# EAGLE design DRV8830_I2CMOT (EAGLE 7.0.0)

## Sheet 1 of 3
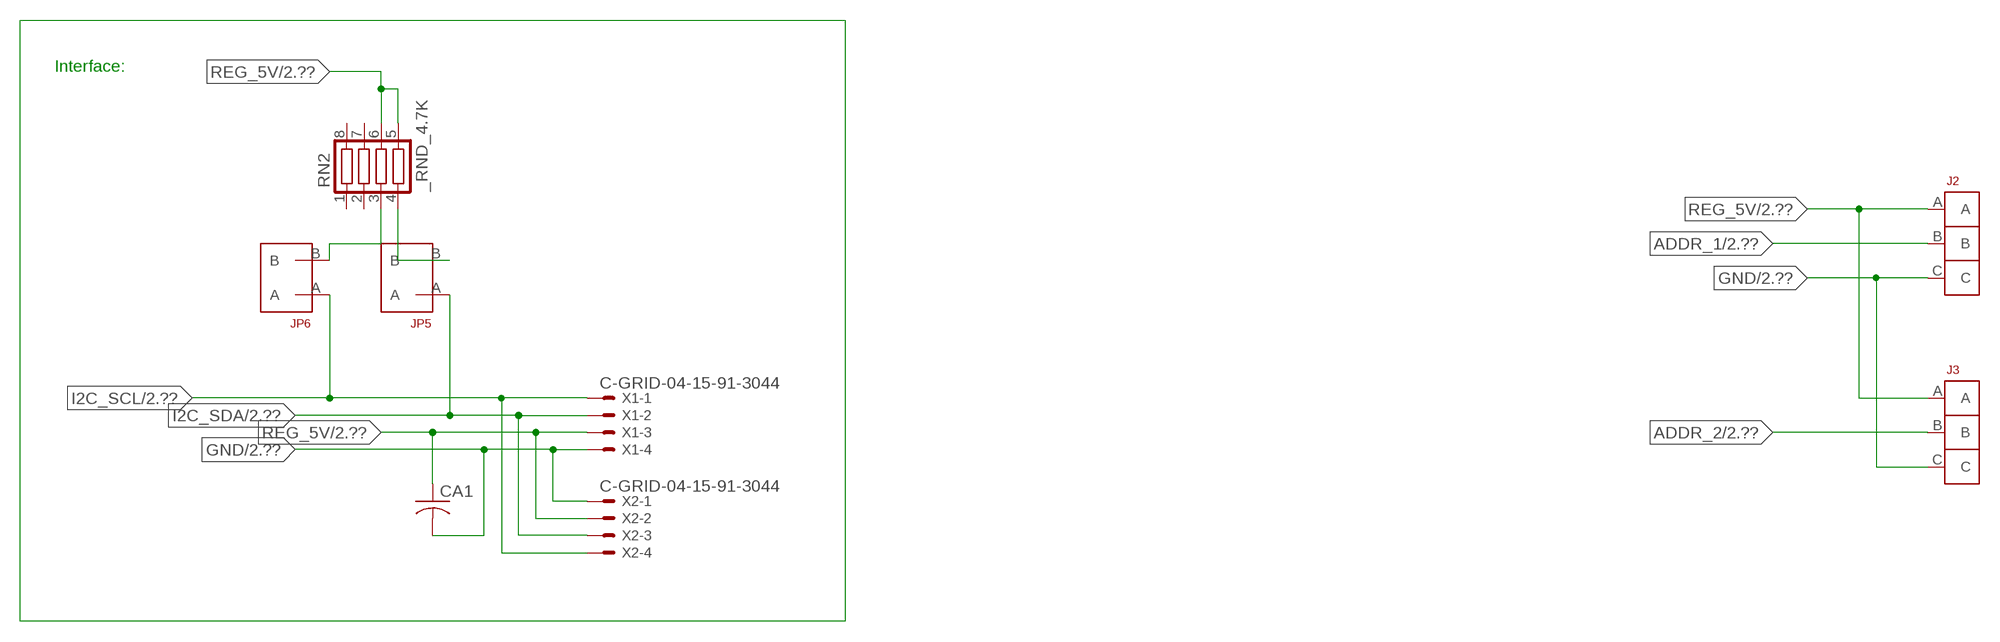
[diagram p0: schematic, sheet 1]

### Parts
CA1  CC1206KRX7R9BB104  [.1UF]
J2  JUMPER_1X3_2MM  [JUMPER_1X3_2MM]
J3  JUMPER_1X3_2MM  [JUMPER_1X3_2MM]
JP5  JUMPER_1X2_2MM  [JUMPER_1X2_2MM]
JP6  JUMPER_1X2_2MM  [JUMPER_1X2_2MM]
RN2  _RND_4.7K  [RND]
X1  C-GRID-04-15-91-3044  [15-91-04]
X2  C-GRID-04-15-91-3044  [15-91-04]

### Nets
ADDR_1: J2.B ; also sheet 2
ADDR_2: J3.B ; also sheet 2
GND: CA1.2 J2.C J3.C X1.4 X2.1 ; also sheet 2,3
I2C_SCL: JP6.A X1.1 X2.4 ; also sheet 2
I2C_SDA: JP5.A X1.2 X2.3 ; also sheet 2
N$1: JP6.B RN2.3
N$2: JP5.B RN2.4
REG_5V: CA1.1 J2.A J3.A RN2.5 RN2.6 X1.3 X2.2 ; also sheet 2,3
Unconnected: RN2.1 RN2.2 RN2.7 RN2.8

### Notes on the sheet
- Interface:

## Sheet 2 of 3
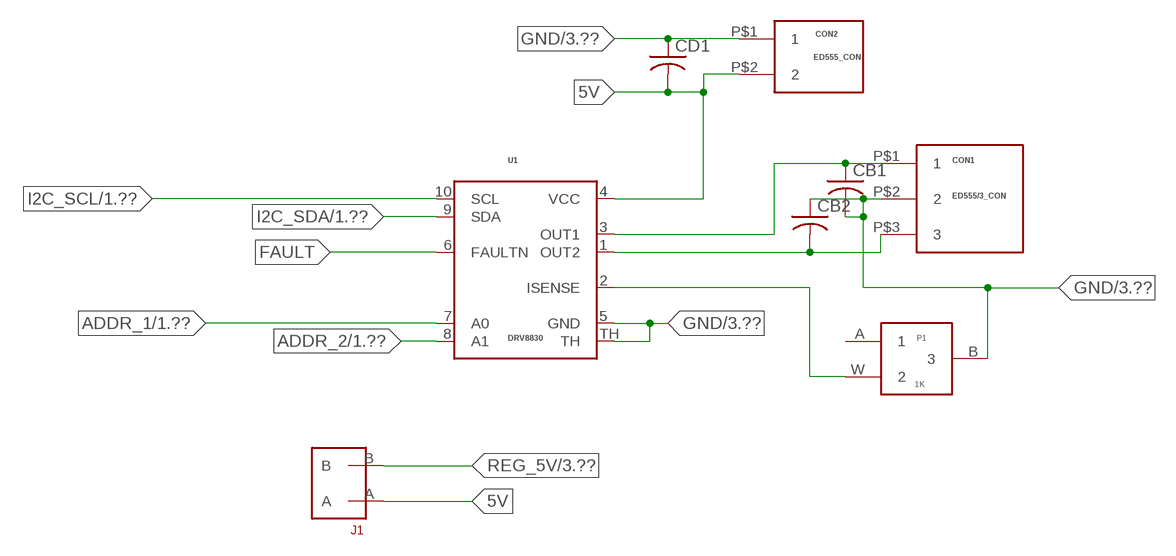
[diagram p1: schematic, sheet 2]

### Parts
CB1  _CB_10UF_25VC1206K  [_CB_10UF_25V]
CB2  _CB_10UF_25VC1206K  [_CB_10UF_25V]
CD1  CC1206KRX7R9BB103C1206K  [CC1206KRX7R9BB103]
CON1  ED555/3_CON  [ED555/3_CON]
CON2  ED555_CON  [ED555_CON]
J1  JUMPER_1X2_2MM  [JUMPER_1X2_2MM]
P1  1K  PW36V  [PW36V]
U1  DRV8830  [10SON]

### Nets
5V: CD1.2 CON2.P$2 J1.A U1.4(VCC)
ADDR_1: U1.7(A0) ; also sheet 1
ADDR_2: U1.8(A1) ; also sheet 1
FAULT: U1.6(FAULTN)
GND: CB1.2 CB2.1 CD1.1 CON1.P$2 CON2.P$1 P1.B U1.5(GND) U1.TH ; also sheet 1,3
I2C_SCL: U1.10(SCL) ; also sheet 1
I2C_SDA: U1.9(SDA) ; also sheet 1
N$3: CB1.1 CON1.P$1 U1.3(OUT1)
N$10: P1.W U1.2(ISENSE)
N$11: CB2.2 CON1.P$3 U1.1(OUT2)
REG_5V: J1.B ; also sheet 1,3
Unconnected: P1.A

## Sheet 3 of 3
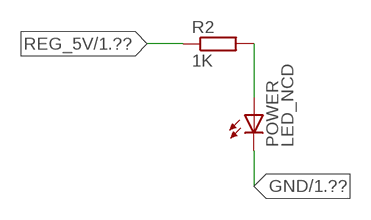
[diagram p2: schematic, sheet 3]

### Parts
POWER  LED_NCD  [CHIPLED_0603]
R2  1K  RESISTOR_SMT-0402  [R402]

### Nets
GND: POWER.C ; also sheet 1,2
N$16: POWER.A R2.2
REG_5V: R2.1 ; also sheet 1,2

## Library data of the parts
CA1 = NCD_ULTIMATE_LIBRARY:CC1206KRX7R9BB104: Capacitor CA .1uF 50V SMT C1206K CC1206KRX7R9BB104
CB1 CB2 = NCD_ULTIMATE_LIBRARY:_CB_10UF_25V: Capacitor 10uF SMT
CD1 = NCD_ULTIMATE_LIBRARY:CC1206KRX7R9BB103: Capacitor CD .01uF SMT CC1206KRX7R9BB103 1206
CON1 = NCD_ULTIMATE_bhaskar:ED555/3_CON: Digikey Con ED1515-ND NCD CON
CON2 = NCD_ULTIMATE_bhaskar:ED555_CON: Digikey ED1514-ND/ ED555/2DS NCD CON
J1 JP5 JP6 = NCD_ULTIMATE_CONNECTORS:JUMPER_1X2_2MM
J2 J3 = NCD_ULTIMATE_CONNECTORS:JUMPER_1X3_2MM
P1 = NCD_ULTIMATE_bhaskar:PW36V: Digikey 490-2889-ND/PV36W503C01B00
POWER = NCD_ULTIMATE_LIBRARY:LED_NCD: LED Digikey 754-1132-2-ND/APT2012SRCPRV
R2 = NCD_ULTIMATE_LIBRARY:RESISTOR_SMT: NCD Resistor
RN2 = NCD_ULTIMATE_LIBRARY:_RND_4.7K: Resistor Array RND SMT 4.7K x 4 Single Resistor Source: http://www.ctscorp.com/components/Datasheets/CTSChipArrayDs.pdf Digikey 742C083472JPTR-ND/742C083472JP; OC_FARNELL: unknown; OC_NEWARK: unknown
U1 = NCD_ULTIMATE_bhaskar:DRV8830: I2C motor driver Digikey 296-28165-2-ND/DRV8830DGQR
X1 X2 = NCD_ULTIMATE_CONNECTORS:C-GRID-04: CONNECTOR 4-Pos I2C wire to board 2.54 mm (0.100") pitch header Digikey WM1342-ND/0015912045; OC_FARNELL: unknown; OC_NEWARK: unknown

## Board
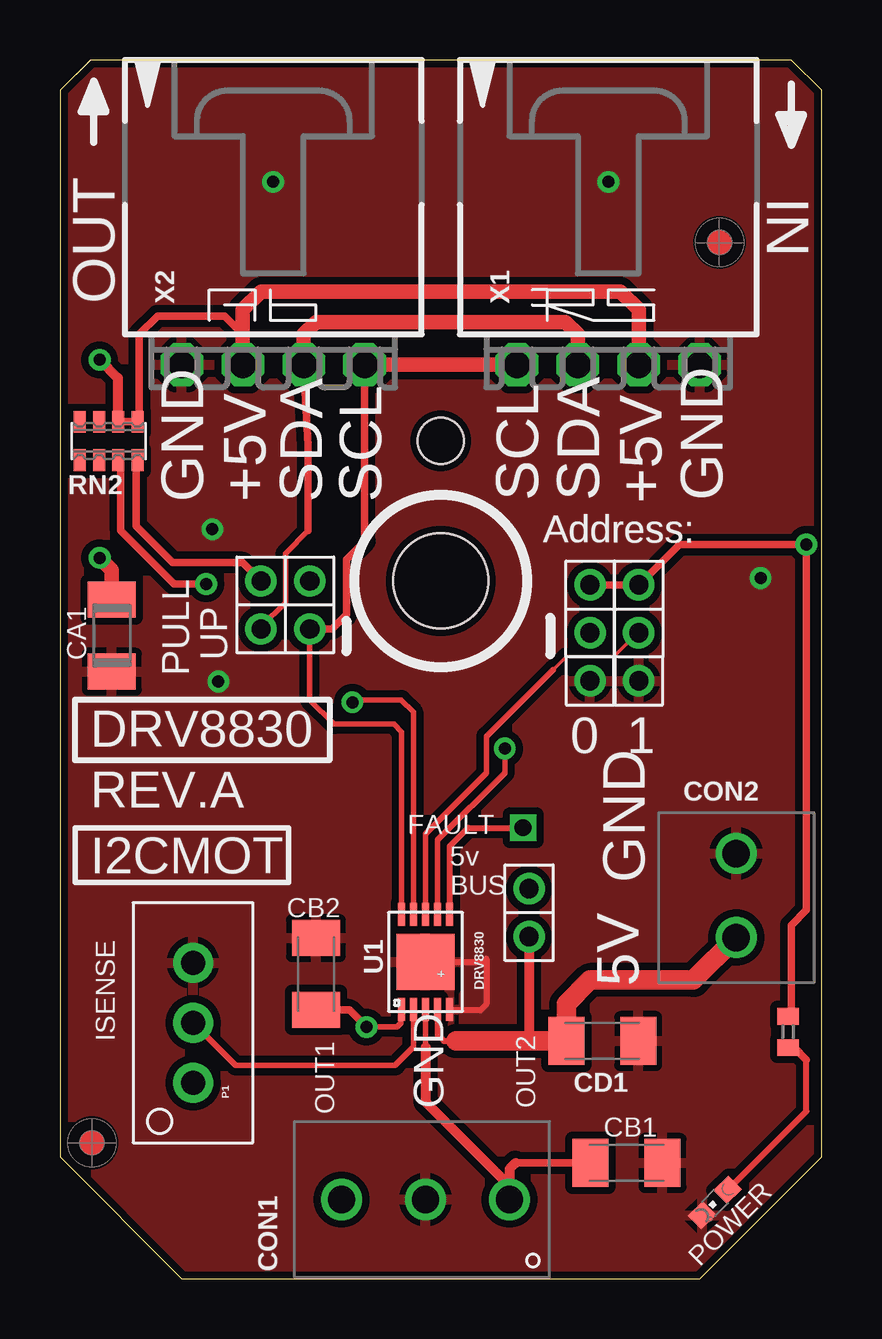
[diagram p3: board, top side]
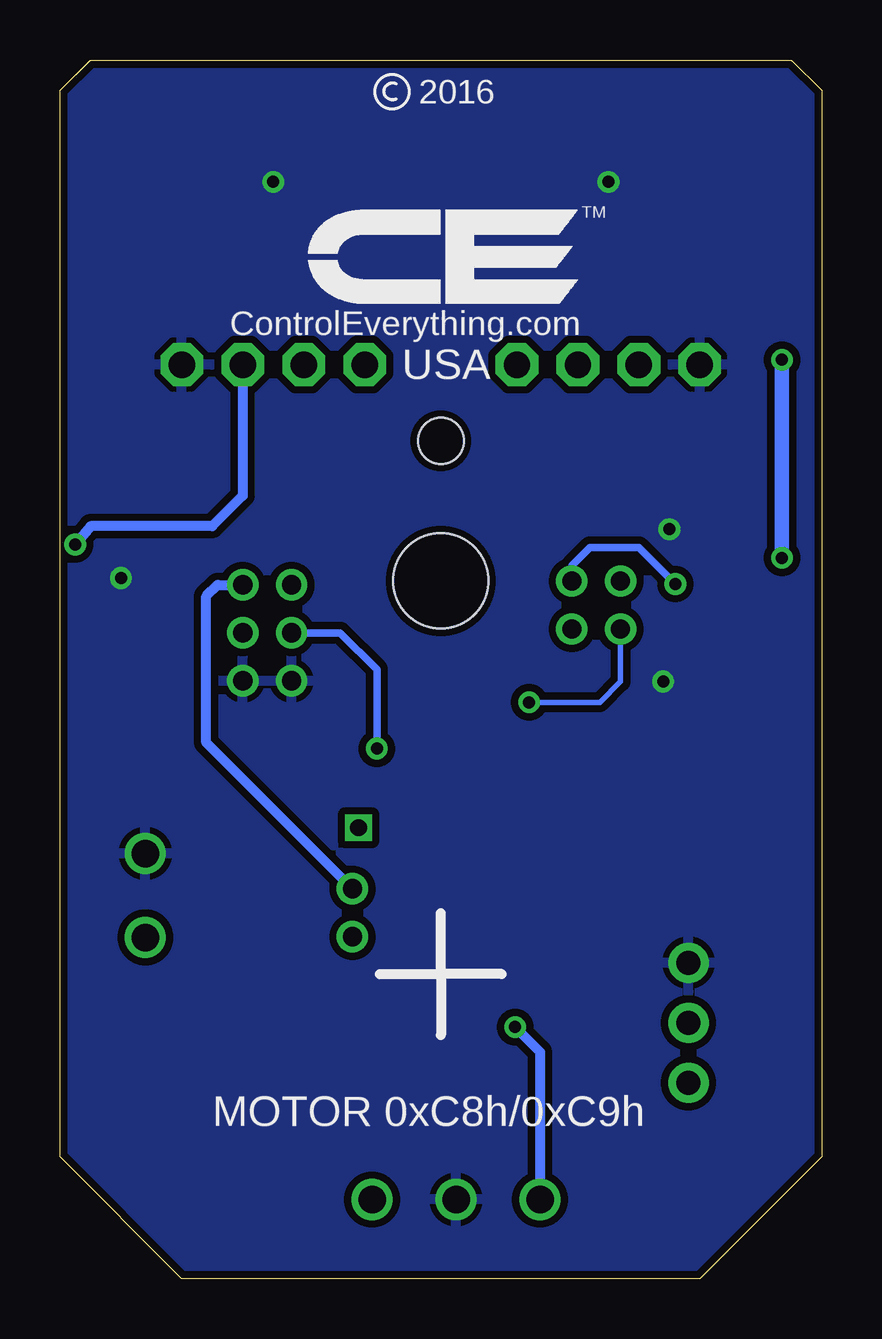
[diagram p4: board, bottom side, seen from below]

Size 31.75 x 50.8 mm. Coordinates in mm from the lower left corner, seen from the top.
Outline: 31.75,5.08 31.75,49.53 30.48,50.8 1.27,50.8 0,49.53 0,5.08 5.08,0 26.67,0 31.75,5.08
Outline: 31.75,5.08 31.75,49.53 30.48,50.8 1.27,50.8 0,49.53 0,5.08 5.08,0 26.67,0 31.75,5.08
Copper layers (1*16): Top 0.035mm / dielectric 1.5mm / Bottom 0.035mm
Design rules "default": minimum track width 5mil, minimum drill 24mil, track to track 5mil, track to pad 5mil, pad to pad 5mil, via to via 5mil, smd to smd 5mil, copper to edge 10mil, drill to drill 8mil, minimum pad ring 10mil, minimum via ring 8mil, stop-mask expansion 2mil, vias tented up to drill 0mil, thermal gap 10mil
Holes 3.96 mm at 15.88,29.08
Holes 1.91 mm at 15.88,34.92

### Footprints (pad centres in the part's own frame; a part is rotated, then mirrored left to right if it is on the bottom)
.1UF = smd 1.5 x 2: 1 -1.5,0; 2 1.5,0
_CB_10UF_25V = smd 1.5 x 2: 1 -1.5,0; 2 1.5,0
CC1206KRX7R9BB103 = smd 1.5 x 2: 1 -1.5,0; 2 1.5,0
ED555/3_CON = drill 1.143: P$1 0,3.5; P$2 0,0; P$3 0,-3.5
ED555_CON = drill 1.143: P$1 0,3.5; P$2 0,0
JUMPER_1X2_2MM = drill 0.8: A 0,2; B 0,0
JUMPER_1X3_2MM = drill 0.8: A 0,2; B 0,0; C 0,-2
PW36V = drill 1 pad 1.676: A -2.5,2.5; B -2.5,-2.5; W -2.5,0
CHIPLED_0603 = smd 0.8 x 0.876: A 0,-0.75; C 0,0.75
R402 = smd 0.7 x 0.9: 1 -0.65,0; 2 0.65,0
RND = smd 0.5 x 0.9: 1 -1.2,-0.8; 2 -0.4,-0.8; 3 0.4,-0.8; 4 1.2,-0.8; 5 1.2,0.8; 6 0.4,0.8; 7 -0.4,0.8; 8 -1.2,0.8
10SON = smd 0.28 x 0.95: 1 -1,-1.475; 2 -0.5,-1.475; 3 0,-1.475; 4 0.5,-1.475; 5 1,-1.475; 6 1,2.491; 7 0.5,2.491; 8 0,2.491; 9 -0.5,2.491; 10 -1,2.491 | smd 2.4 x 2.35: TH 0,0.508
15-91-04 = drill 1.1 pad 1.778 octagon: 1 -3.81,-7.62; 2 -1.27,-7.62; 3 1.27,-7.62; 4 3.81,-7.62

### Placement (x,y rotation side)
CA1  2.16,26.81 270 top
CB1  23.62,4.83 0 top
CB2  10.67,12.7 270 top
CD1  22.61,9.91 180 top
CON1  15.24,3.3 270 top
CON2  28.19,14.22 0 top
J1  19.56,16.26 180 top
J2  22.1,26.92 0 top
J3  24.13,26.92 0 top
JP5  8.38,29.08 180 top
JP6  10.41,29.08 180 top
P1  3.05,10.67 180 top
POWER  27.3,3.18 135 top
R2  30.35,10.29 270 top
RN2  2.03,34.92 0 top
U1  15.24,12.7 0 top
U$5  [VISION_REF10]  1.33,5.66 90 top
U$28  [VISION_REF10]  27.5,43.19 90 top
X1  22.86,45.72 0 top
X2  8.89,45.72 0 top

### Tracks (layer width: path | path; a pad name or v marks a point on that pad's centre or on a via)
5V
  Top 0.229: U1.4
  Top 0.254: U1.4 15.75,10.16 16,9.91 16.51,9.91
  Top 0.406: J1.A 19.56,9.91
  Top 0.813: 16.51,9.91 19.56,9.91 CD1.2 21.11,11.45 22.1,12.45 26.42,12.45 CON2.P$2
ADDR_1  (via drill 0.5)
  Top 0.229: v18.54,22.1 18.54,21.08 15.74,18.28 U1.7
  Bottom 0.305: v18.54,22.1 18.54,25.4 20.07,26.92 J2.B
ADDR_2
  Top 0.152: 20.57,25.4 21.11,25.93 23.09,25.93 24.08,26.92 J3.B
  Top 0.229: U1.8 15.24,18.54 17.78,21.08 17.78,22.61 20.57,25.4
FAULT  (via drill 0.7)
  Top 0.254: U1.6 16.26,15.21 16.26,18.03 17.02,18.8 v19.3,18.8
GND  (via drill 0.5)
  Top 0.254: U1.TH 17.65,13.21 17.78,13.34 17.78,11.43 17.53,11.18 16.29,11.18 U1.5
  other vias: 8.89,45.72 22.86,45.72 6.35,31.24 6.6,24.89 29.21,29.21
  pour Bottom (isolate 0.305): 4.45,-0.63 -0.64,4.45 -0.64,50.17 0.64,51.44 31.11,51.44 32.38,50.17 32.38,4.45 27.3,-0.63
  pour Top (isolate 0.305): 3.81,-1.27 -1.27,3.81 -1.27,50.8 0,52.07 31.75,52.07 33.02,50.8 33.02,3.81 27.94,-1.27
I2C_SCL
  Top 0.229: U1.10 14.24,22.79 13.92,23.11 11.43,23.11 10.41,24.13 JP6.A
  Top 0.305: X2.4 12.7,30.73 11.94,29.97 11.94,27.69 11.34,27.08 JP6.A
  Top 0.61: X2.4 X1.1
I2C_SDA  (via drill 0.5)
  Top 0.229: U1.9 14.74,22.75 14.73,23.27 14.73,23.62 14.22,24.13 12.19,24.13 | 10.35,31.18 9.4,30.23 9.4,28.19 8.38,27.18 JP5.A
  Top 0.305: 10.35,31.18 10.35,34.73 X2.3 | v12.19,24.03 12.19,24.13
  Top 0.61: X2.3 10.16,39.37 10.67,39.88 21.08,39.88 21.59,39.37 X1.2
  Bottom 0.229: JP5.A 8.38,24.89 9.25,24.03 v12.19,24.03
N$1  (via drill 0.5)
  Top 0.305: RN2.3 2.54,34.02 2.54,31.18 4.76,28.96 v6.1,28.96
  Bottom 0.305: v6.1,28.96 7.62,30.48 9.65,30.48 10.41,29.72 JP6.B
N$2
  Top 0.305: RN2.4 3.17,34.07 3.17,31.37 4.7,29.85 7.62,29.85 JP5.B
N$3
  Top 0.229: U1.3 15.24,9.65
  Top 0.305: 18.99,4.83 CB1.1
  Top 0.406: 15.24,9.65 15.24,7.37 18.74,3.87 | 18.74,3.87 18.74,3.81 CON1.P$1 | 18.99,4.83 18.74,4.57 18.74,3.87
N$10
  Top 0.229: P1.W 7.33,8.89 13.97,8.89 14.74,9.66 U1.2
N$11  (via drill 0.5)
  Top 0.229: v12.78,10.49 14.05,10.49 14.22,10.67 14.22,11.21 U1.1
  Top 0.305: v12.78,10.49 12.07,11.2 CB2.2
  Bottom 0.305: v12.78,10.49 12.75,10.47
  Bottom 0.406: 12.75,10.47 11.74,9.45 CON1.P$3
N$16
  Top 0.254: POWER.A 31.11,6.99 31.11,9.13
  Top 0.305: 31.11,9.13 30.61,9.64 R2.2
REG_5V  (via drill 0.5)
  Top 0.305: 7.62,39.37 7.49,39.37 | RN2.6 RN2.5 3.3,35.8 3.3,39.37 4.06,40.13 6.86,40.13 7.62,39.37 | X2.2 7.62,39.37 | J2.A J3.A 25.81,30.61 v31.11,30.61 31.11,15.37 30.48,14.73 30.48,11.06 R2.1
  Top 0.406: v1.65,38.3 2.41,37.54 2.41,35.74 RN2.6
  Top 0.61: X2.2 7.62,40.39 8.38,41.15 23.37,41.15 24.13,40.39 X1.3 | CA1.1 2.16,29.54 v1.65,30.05
  Bottom 0.406: X1.3 24.13,32.64 25.4,31.37 30.48,31.37 v31.11,30.61 | J1.B 25.65,22.35 25.65,28.45 25.18,28.92 J3.A | X1.3
  Bottom 0.61: v1.65,30.05 v1.65,38.3

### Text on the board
tPlace: I2CMOT | OUT1 | OUT2
tNames: IN | OUT | GND | GND | +5V | +5V | SDA | SDA | SCL | SCL | SCL | SCL | SDA | SDA | +5V | +5V | GND | GND | Address: | Address: | UP | PULL | DRV8830 | 0 | 1 | REV.A | FAULT | GND | 5v / BUS | 5V | ISENSE | GND
bNames: 2016 | TM | ControlEverything.com | USA | MOTOR 0xC8h/0xC9h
